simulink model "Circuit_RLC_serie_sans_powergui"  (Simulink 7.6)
settings: Solver=ode23t  StartTime=0.0  StopTime=0.04  RelTol=1e-3
libraries: powerlib x8

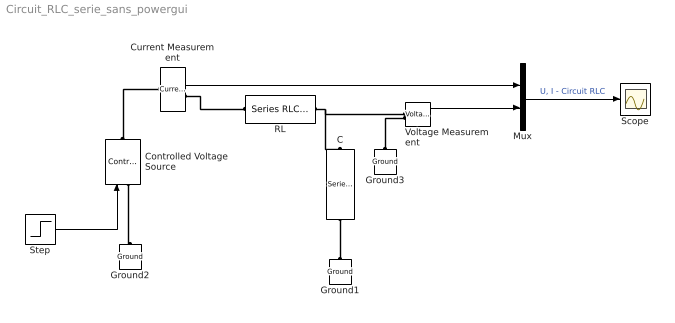
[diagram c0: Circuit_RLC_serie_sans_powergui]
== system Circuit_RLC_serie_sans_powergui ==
  C : powerlib/Elements/Series RLC Branch  DialogController=POWERSYS.PowerSysDialog  PhysicalDomain=powersysdomain  SubClassName=unknown  LeftPortType=p1  RightPortType=p1  LConnTagsString=__new0  RConnTagsString=__new0  BranchType=C  Resistance=1  Inductance=1e-3  SetiL0=off  InitialCurrent=0  Capacitance=0.001  Setx0=off  InitialVoltage=0  Measurements=None
  Controlled Voltage Source : powerlib/Electrical Sources/Controlled Voltage Source  DialogController=POWERSYS.PowerSysDialog  SystemSampleTime=-1  Initialize=on  Source_Type=AC  Amplitude=0  Phase=0  Frequency=0  Measurements=None
  Current Measurement : powerlib/Measurements/Current Measurement  DialogController=POWERSYS.PowerSysDialog  SystemSampleTime=-1  PhasorSimulation=off  OutputType=Complex  PSBequivalent=0
  Ground1 : powerlib/Elements/Ground  DialogController=POWERSYS.PowerSysDialog  PhysicalDomain=powersysdomain  SubClassName=unknown  LeftPortType=p1  RightPortType=p1  LConnTagsString=a
  Ground2 : powerlib/Elements/Ground  DialogController=POWERSYS.PowerSysDialog  PhysicalDomain=powersysdomain  SubClassName=unknown  LeftPortType=p1  RightPortType=p1  LConnTagsString=a
  Ground3 : powerlib/Elements/Ground  DialogController=POWERSYS.PowerSysDialog  PhysicalDomain=powersysdomain  SubClassName=unknown  LeftPortType=p1  RightPortType=p1  LConnTagsString=a
  Mux : Mux  Inputs=2
  RL : powerlib/Elements/Series RLC Branch  DialogController=POWERSYS.PowerSysDialog  PhysicalDomain=powersysdomain  SubClassName=unknown  LeftPortType=p1  RightPortType=p1  LConnTagsString=__new0  RConnTagsString=__new0  BranchType=RL  Resistance=4  Inductance=10e-3  SetiL0=off  InitialCurrent=0  Capacitance=0  Setx0=off  InitialVoltage=0  Measurements=None
  Scope : Scope
  Step : Step  Time=0  SampleTime=0
  Voltage Measurement : powerlib/Measurements/Voltage Measurement  DialogController=POWERSYS.PowerSysDialog  SystemSampleTime=-1  PhasorSimulation=off  OutputType=Complex  PSBequivalent=0
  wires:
  Voltage Measurement/1 -> Mux/2
  Current Measurement/1 -> Mux/1
  Step/1 -> Controlled Voltage Source/1
  Mux/1 -> Scope/1  "U, I - Circuit RLC"
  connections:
  Current Measurement/RConn1 -- RL/LConn1
  RL/RConn1 -- C/LConn1 -- Voltage Measurement/LConn1
  C/RConn1 -- Ground1/LConn1
  Controlled Voltage Source/RConn1 -- Current Measurement/LConn1
  Controlled Voltage Source/LConn1 -- Ground2/LConn1
  Ground3/LConn1 -- Voltage Measurement/LConn2
